FUNCTION FC 53 : VOID
TITLE =
VERSION : 0.1

BEGIN
NETWORK
TITLE =Part in die
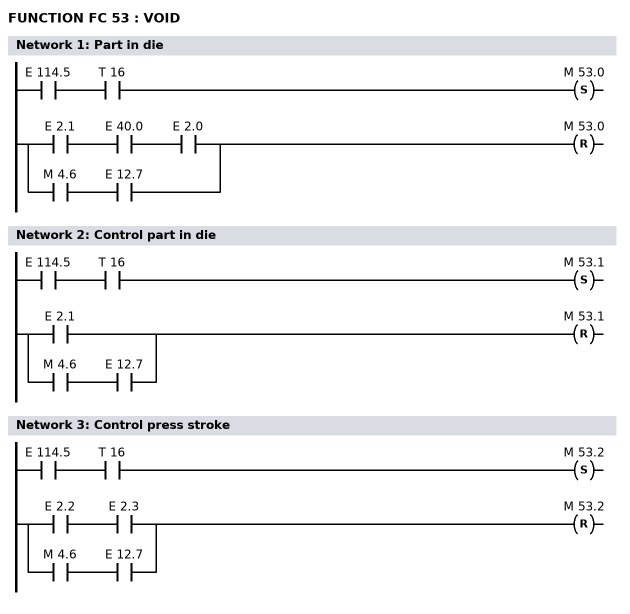
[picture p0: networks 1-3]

      U     E    114.5;
      U     T     16;
      S     M     53.0;
      U(    ;
      U     E      2.1;
      U     E     40.0;
      U     E      2.0;
      O     ;
      U     M      4.6;
      U     E     12.7;
      )     ;
      R     M     53.0;
      NOP   0;
NETWORK
TITLE =Control part in die

      U     E    114.5;
      U     T     16;
      S     M     53.1;
      U(    ;
      O     E      2.1;
      O     ;
      U     M      4.6;
      U     E     12.7;
      )     ;
      R     M     53.1;
      NOP   0;
NETWORK
TITLE =Control press stroke

      U     E    114.5;
      U     T     16;
      S     M     53.2;
      U(    ;
      U     E      2.2;
      U     E      2.3;
      O     ;
      U     M      4.6;
      U     E     12.7;
      )     ;
      R     M     53.2;
      NOP   0;
END_FUNCTION

